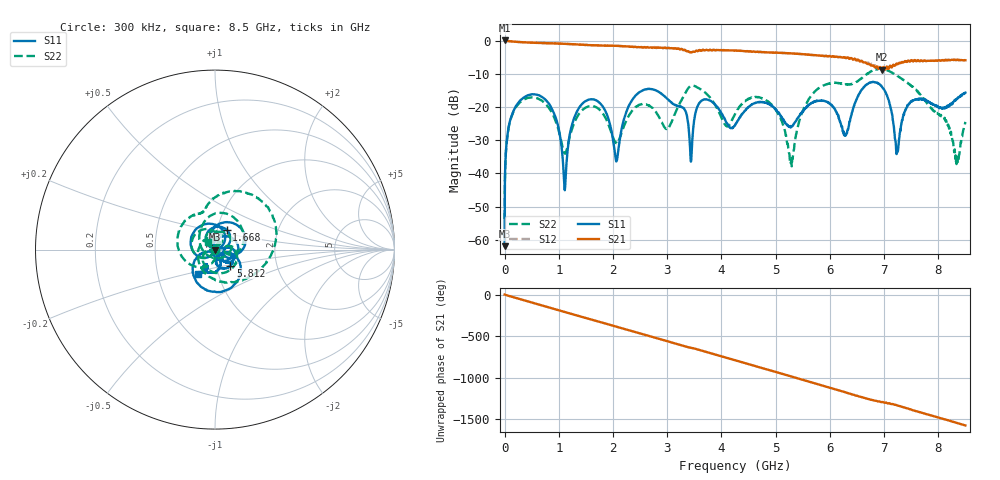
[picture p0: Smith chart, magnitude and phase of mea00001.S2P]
!Agilent Technologies,E5071B,MY42402595,A.08.01
!Date: Tue Jan 02 10:10:52 2001
!Data & Calibration Information:
!Freq	S11:SOLT2(ON)	S21:SOLT2(ON)	S12:SOLT2(ON)	S22:SOLT2(ON)
# Hz S dB R 50
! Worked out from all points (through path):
!   1601 points, 300 kHz to 8.5 GHz, reference 50 ohm
!   highest |S21| = 0.02 dB at 300 kHz (marker M1); lowest = -8.8 dB at 6.959 GHz (marker M2)
!   group delay of S21, straight-line fit = 514 ps
!   lowest |S11| = -61.9 dB at 300 kHz (marker M3), VSWR 1.00, Z = 50 - j0.0768 ohm
!   |S11| at or under -10 dB: start of sweep to end of sweep
!   |S22| runs from -53.7 to -8.4 dB; largest |S21 - S12| = 0.033
!   S11 on the Smith chart (normalised r, x): 300 kHz: 1.00, -0.00; 1.668 GHz: 1.11, +0.25; 5.812 GHz: 1.17, -0.21; 8.5 GHz: 0.80, -0.22
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300000  -61.91 -73.0  0.02 0.1  -0.02 -0.3  -53.75 -124.7
6.404775e7  -27.20 -126.7  -0.17 -13.3  -0.15 -13.3  -27.25 -126.1
2.499787e8  -18.83 -168.5  -0.43 -48.9  -0.42 -48.9  -19.24 -163.7
8.874562e8  -21.04 50.4  -0.86 -168.1  -0.84 -168.1  -22.22 78.6
1.110573e9  -45.07 91.4  -0.98 150.0  -0.99 150.0  -34.03 107.0
1.418687e9  -19.29 110.1  -1.28 92.4  -1.27 92.6  -21.20 126.3
1.668366e9  -17.88 59.9  -1.45 46.4  -1.45 46.6  -19.94 82.3
2.061477e9  -36.41 58.9  -1.60 -26.6  -1.60 -26.7  -30.80 75.8
2.316468e9  -18.92 95.5  -1.87 -74.6  -1.89 -74.5  -21.99 96.4
2.837075e9  -15.39 9.4  -2.15 -170.7  -2.00 -171.4  -22.67 -23.7
3.341745e9  -21.45 -48.7  -3.05 92.2  -3.03 92.8  -15.63 111.2
3.830477e9  -18.51 -15.4  -2.92 8.4  -2.90 8.6  -17.95 -6.8
4.25015e9  -25.49 2.6  -3.03 -71.0  -3.03 -71.2  -22.20 15.9
4.855754e9  -18.97 -36.6  -3.59 175.2  -3.57 175.1  -18.32 -102.7
5.286051e9  -25.88 -30.3  -3.86 94.0  -3.89 93.8  -36.25 -134.4
5.668537e9  -18.80 -29.9  -4.32 21.1  -4.36 21.2  -16.33 -143.5
5.81197e9  -18.12 -46.2  -4.52 -6.2  -4.56 -5.8  -14.18 -173.9
6.959429e9  -13.91 -122.2  -8.82 146.2  -8.22 144.4  -8.52 35.7
7.086925e9  -18.04 -152.8  -8.44 131.6  -8.10 128.6  -9.15 11.9
7.240982e9  -33.57 -117.5  -7.00 104.6  -7.14 104.6  -10.58 -14.6
7.782838e9  -18.06 -118.5  -6.20 -0.1  -6.13 0.3  -18.67 -139.0
8.5e9  -15.68 -124.8  -5.93 -136.3  -5.92 -137.1  -24.50 131.2
